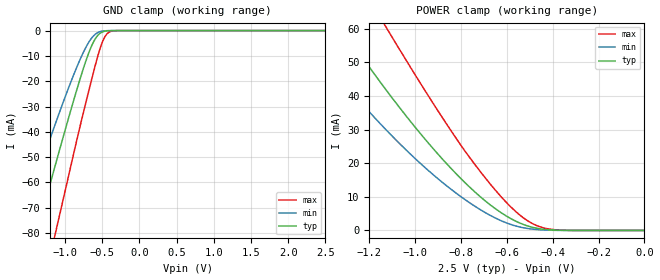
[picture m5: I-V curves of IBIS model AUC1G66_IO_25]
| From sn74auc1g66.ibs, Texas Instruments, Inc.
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[Model]   AUC1G66_IO_25
Model_type  Terminator
| variable   typ   min   max
C_comp   2.75pF   2.51pF   2.89pF
| C_tri-state   2.75pF   2.51pF   2.89pF
[Temperature Range]   40   100   -40
| Ambient temperature   25   85   -40
[Voltage range]   2.5   2.3   2.7
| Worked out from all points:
|   GND clamp passes 1 mA (typ) near -0.53 V on its own axis
|   POWER clamp passes 1 mA (typ) near -0.49 V on its own axis
[GND Clamp]
| AUC1G66_IO_25
|   Voltage   I(typ)   I(min)   I(max)
-2.7V     -221.8mA   -178.5mA   -275mA
-1.62V    -105.6mA   -79.27mA   -141.7mA
-1.37V    -78.59mA   -57.12mA   -110.4mA
-1.13V    -52.92mA   -36.7mA    -79.94mA
-1.1V     -49.75mA   -34.24mA   -76.11mA
-900mV    -29.05mA   -18.56mA   -50.5mA
-765mV    -15.92mA   -9.224mA   -33.67mA
-650mV    -6.462mA   -3.219mA   -20.08mA
-560mV    -1.882mA   -771.5uA   -10.03mA
-465mV    -242.2uA   -89.82uA   -2.444mA
-355mV    -11.13uA   -5.239uA   -117.8uA
2.5V      617.7pA    256.6nA    637.3pA
[POWER Clamp]
| AUC1G66_IO_25
|   Voltage   I(typ)   I(min)   I(max)
-2.7V     217.7mA    187.7mA    248.3mA
-1.49V    77.66mA    59.08mA    102.8mA
-1.32V    60.26mA    44.66mA    82.76mA
-1.13V    42.11mA    30.16mA    60.84mA
-1.105V   39.85mA    28.4mA     58.01mA
-935mV    25.42mA    17.4mA     39.25mA
-790mV    14.73mA    9.55mA     24.33mA
-645mV    6.229mA    3.535mA    11.58mA
-530mV    1.841mA    833.9uA    3.874mA
-470mV    668.2uA    277.2uA    1.462mA
-390mV    106.5uA    46.38uA    213.7uA
-35.59fV  617.7pA    929.9pA    792.6pA
